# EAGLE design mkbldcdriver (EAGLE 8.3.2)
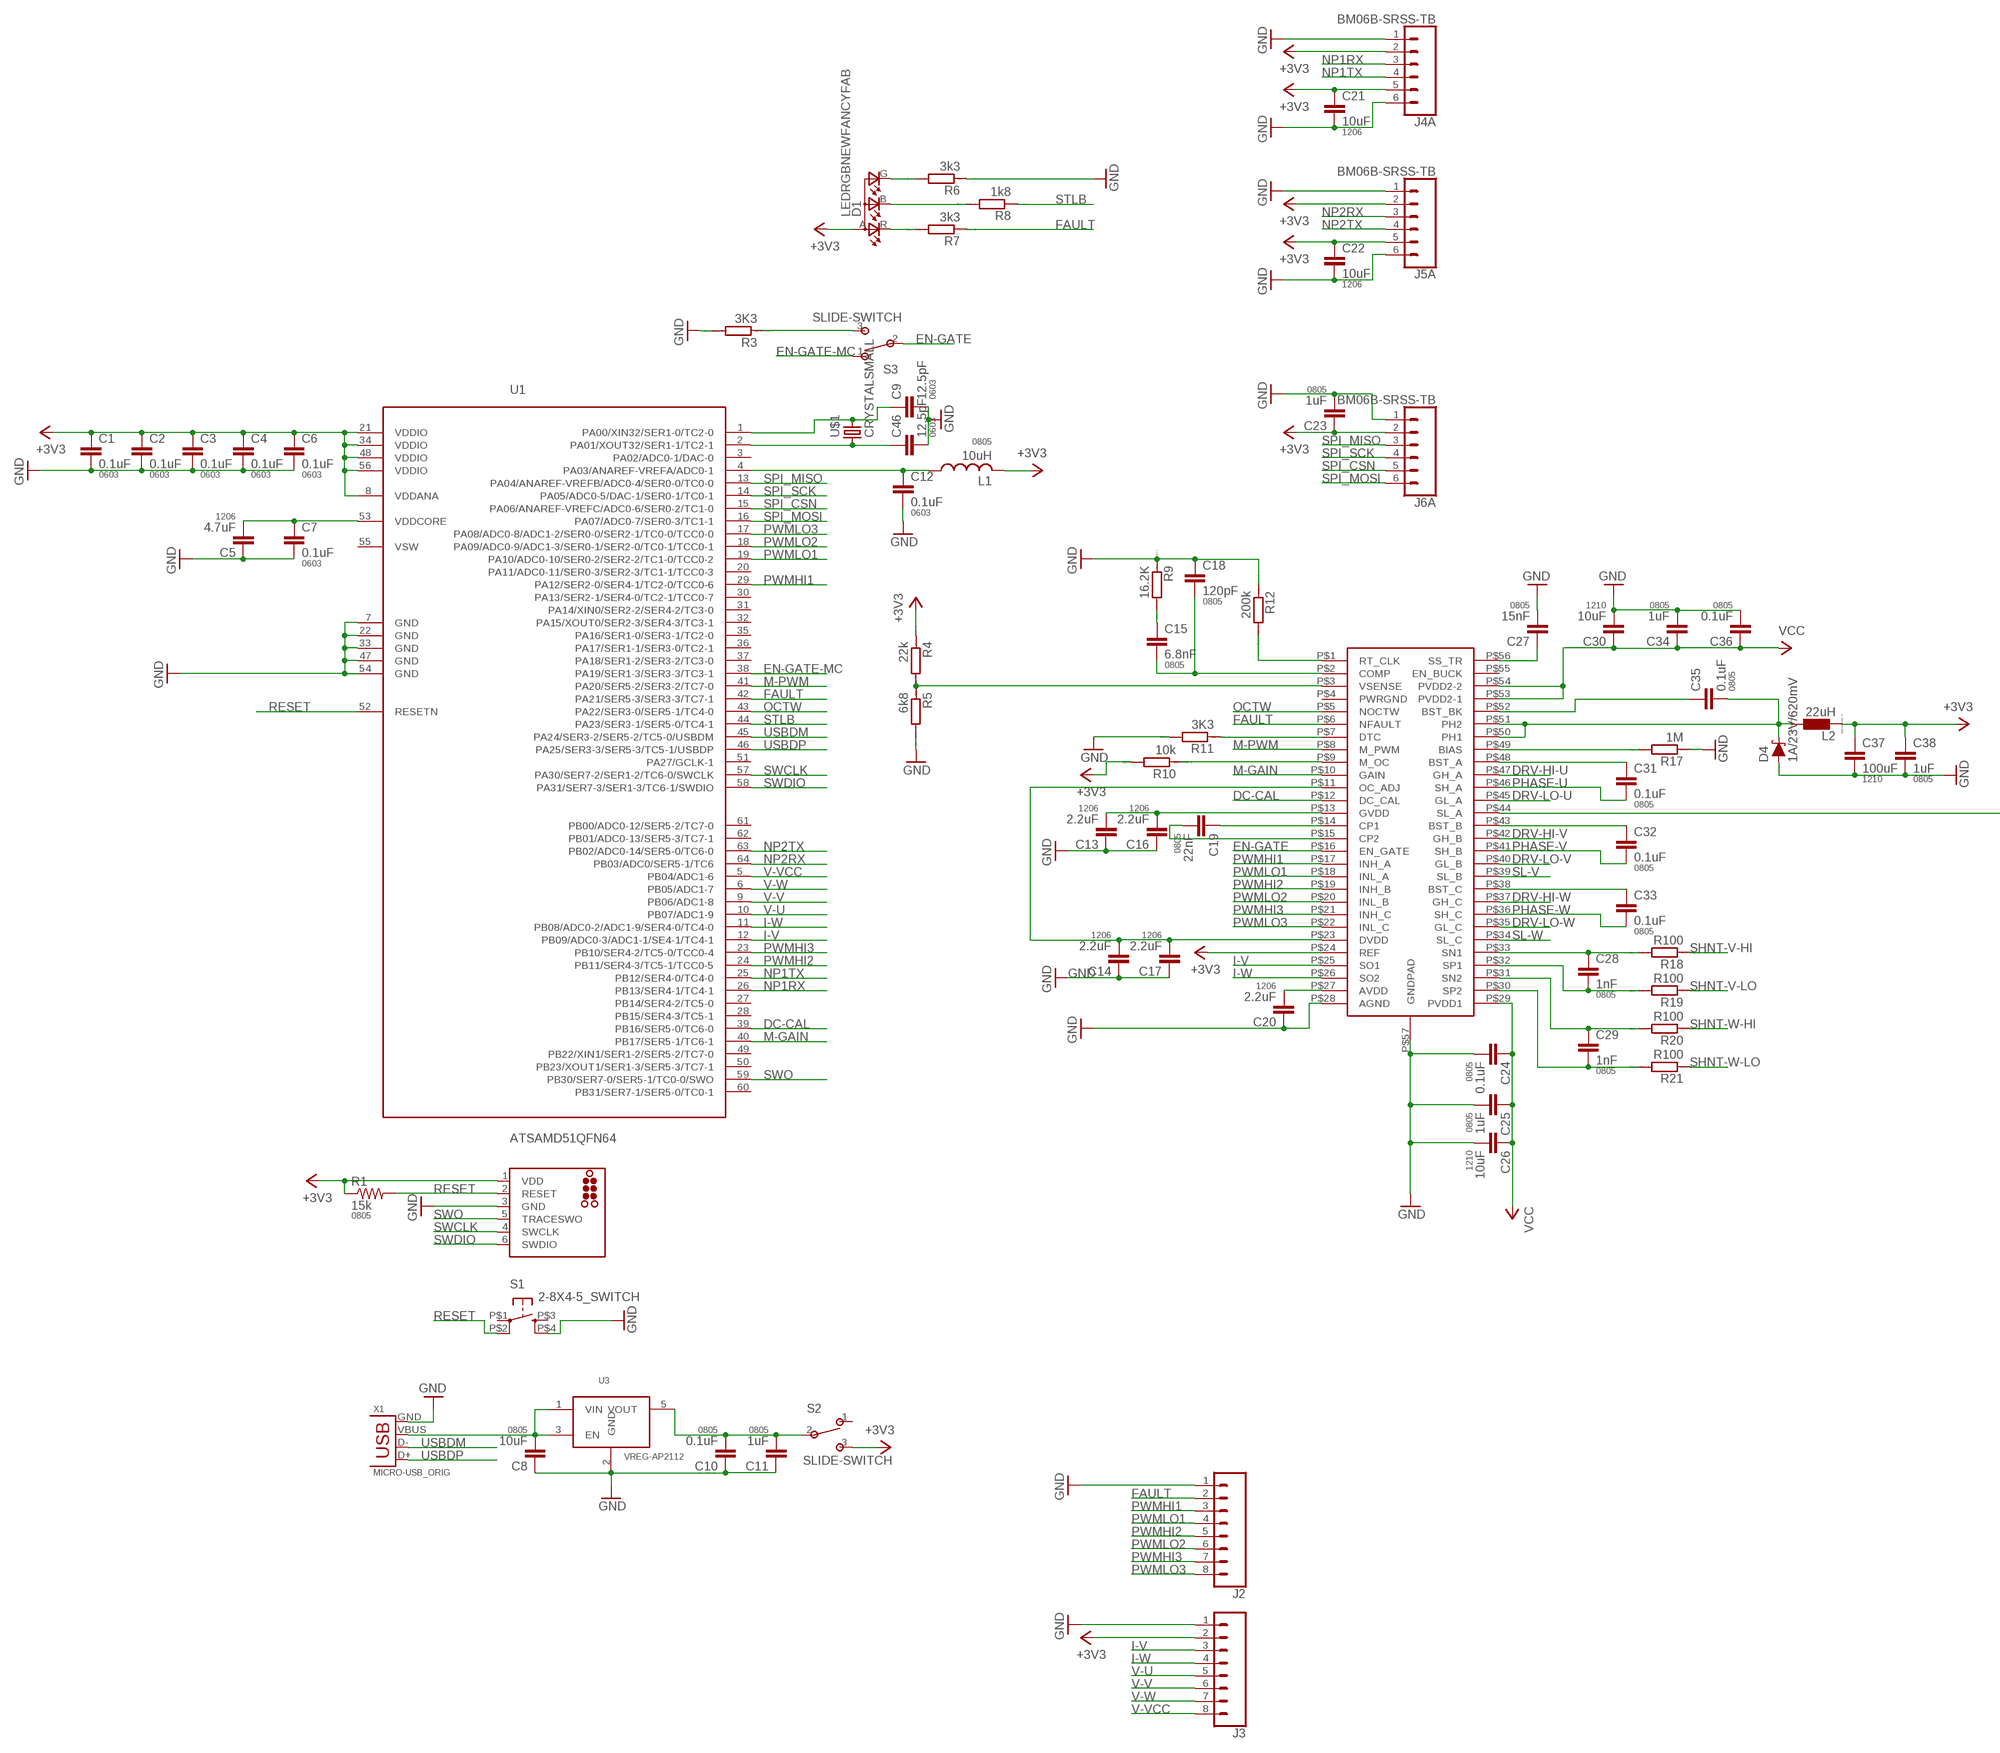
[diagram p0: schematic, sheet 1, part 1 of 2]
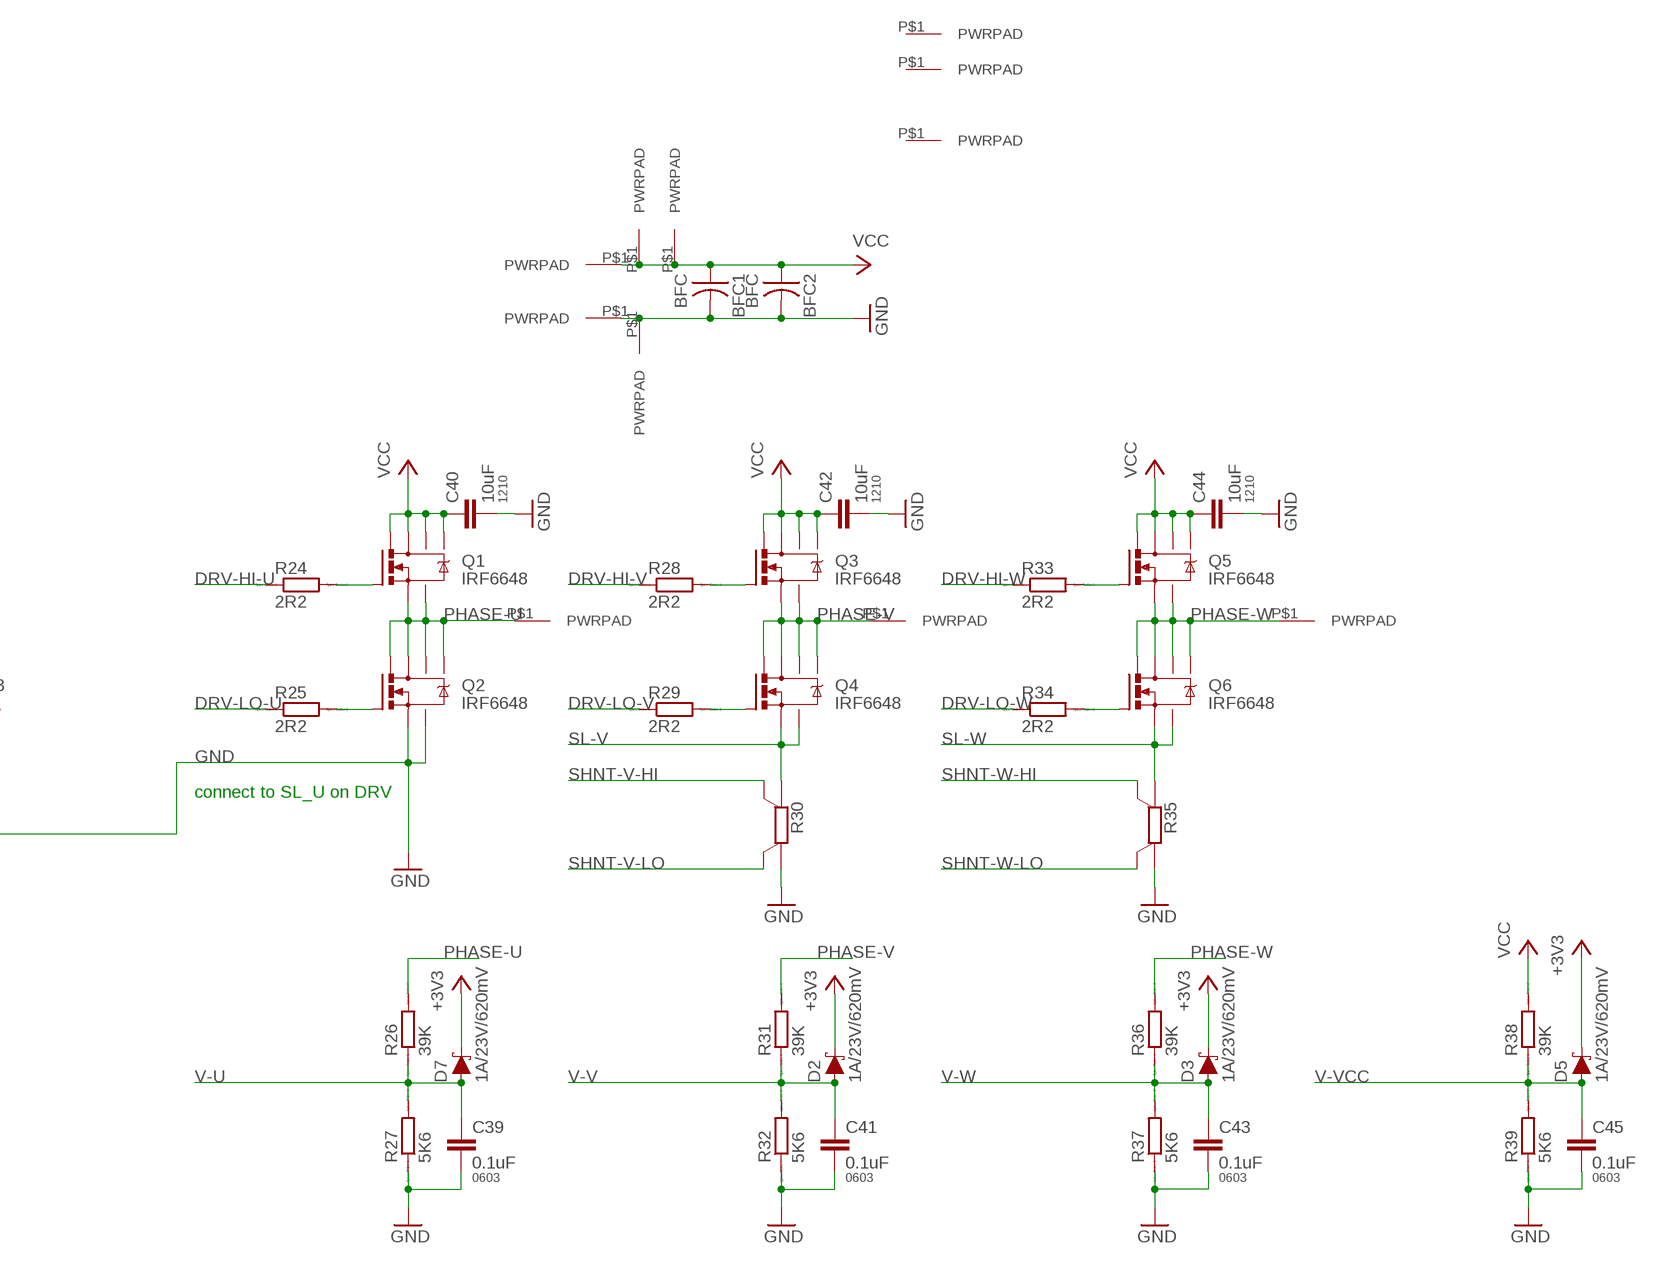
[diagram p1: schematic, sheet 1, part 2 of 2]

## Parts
BFC1  BFC  [BFC]
BFC2  BFC  [BFC]
C1  0.1uF  CAP0603-CAP  [0603-CAP]
C2  0.1uF  CAP0603-CAP  [0603-CAP]
C3  0.1uF  CAP0603-CAP  [0603-CAP]
C4  0.1uF  CAP0603-CAP  [0603-CAP]
C5  4.7uF  CAP1206  [1206]
C6  0.1uF  CAP0603-CAP  [0603-CAP]
C7  0.1uF  CAP0603-CAP  [0603-CAP]
C8  10uF  CAP0805  [0805]
C9  12.5pF  CAP0603-CAP  [0603-CAP]
C10  0.1uF  CAP0805  [0805]
C11  1uF  CAP0805  [0805]
C12  0.1uF  CAP0603-CAP  [0603-CAP]
C13  2.2uF  CAP1206  [1206]
C14  2.2uF  CAP1206  [1206]
C15  6.8nF  CAP0805  [0805]
C16  2.2uF  CAP1206  [1206]
C17  2.2uF  CAP1206  [1206]
C18  120pF  CAP0805  [0805]
C19  22nF  CAP0805  [0805]
C20  2.2uF  CAP1206  [1206]
C21  10uF  CAP1206  [1206]
C22  10uF  CAP1206  [1206]
C23  1uF  CAP0805  [0805]
C24  0.1uF  CAP0805  [0805]
C25  1uF  CAP0805  [0805]
C26  10uF  CAP1210  [1210]
C27  15nF  CAP0805  [0805]
C28  1nF  CAP0805  [0805]
C29  1nF  CAP0805  [0805]
C30  10uF  CAP1210  [1210]
C31  0.1uF  CAP0805  [0805]
C32  0.1uF  CAP0805  [0805]
C33  0.1uF  CAP0805  [0805]
C34  1uF  CAP0805  [0805]
C35  0.1uF  CAP0805  [0805]
C36  0.1uF  CAP0805  [0805]
C37  100uF  CAP1210  [1210]
C38  1uF  CAP0805  [0805]
C39  0.1uF  CAP0603-CAP  [0603-CAP]
C40  10uF  CAP1210  [1210]
C41  0.1uF  CAP0603-CAP  [0603-CAP]
C42  10uF  CAP1210  [1210]
C43  0.1uF  CAP0603-CAP  [0603-CAP]
C44  10uF  CAP1210  [1210]
C45  0.1uF  CAP0603-CAP  [0603-CAP]
C46  12.5pF  CAP0603-CAP  [0603-CAP]
D1  LEDRGBNEWFANCYFAB  [P-LCC-4-FANCYFAB]
D2  1A/23V/620mV  DIODE-SCHOTTKY-BAT20J  [SOD-323]
D3  1A/23V/620mV  DIODE-SCHOTTKY-BAT20J  [SOD-323]
D4  1A/23V/620mV  DIODE-SCHOTTKY-BAT20J  [SOD-323]
D5  1A/23V/620mV  DIODE-SCHOTTKY-BAT20J  [SOD-323]
D7  1A/23V/620mV  DIODE-SCHOTTKY-BAT20J  [SOD-323]
J1  TC2030-SWD-MCP  [TC2030-MCP]
J2  CONN_08NO_SILK_FEMALE_PTH  [1X08_NO_SILK]
J3  CONN_08NO_SILK_FEMALE_PTH  [1X08_NO_SILK]
J4  BM06B-SRSS-TB  JST_6_PIN_HORIZONTAL  [JST-6-SMD-HORI-1.0MM]
J5  BM06B-SRSS-TB  JST_6_PIN_HORIZONTAL  [JST-6-SMD-HORI-1.0MM]
J6  BM06B-SRSS-TB  JST_6_PIN_HORIZONTAL  [JST-6-SMD-HORI-1.0MM]
J7  PWRPAD2-5MM  [PWRPAD_2-5MM]
J8  PWRPADM3  [PWRPAD_3-25MM]
J9  PWRPADM3  [PWRPAD_3-25MM]
J10  PWRPADM3  [PWRPAD_3-25MM]
J11  PWRPADM3  [PWRPAD_3-25MM]
J12  PWRPADM3  [PWRPAD_3-25MM]
J13  PWRPADM3  [PWRPAD_3-25MM]
J14  PWRPADM3  [PWRPAD_3-25MM]
J15  PWRPADM3  [PWRPAD_3-25MM]
J16  PWRPAD2-5MM  [PWRPAD_2-5MM]
J17  PWRPAD2-5MM  [PWRPAD_2-5MM]
L1  10uH  INDUCTOR-0805  [0805]
L2  22uH  L  [L1812]
Q1  IRF6648  [DIRECTFET]
Q2  IRF6648  [DIRECTFET]
Q3  IRF6648  [DIRECTFET]
Q4  IRF6648  [DIRECTFET]
Q5  IRF6648  [DIRECTFET]
Q6  IRF6648  [DIRECTFET]
R1  15k  RESISTOR0805-RES  [0805]
R3  3K3  R  [R0805]
R4  22k  R  [R0805]
R5  6k8  R  [R0805]
R6  3k3  R  [R0805]
R7  3k3  R  [R0805]
R8  1k8  R  [R0805]
R9  16.2K  R  [R0805]
R10  10k  R  [R0805]
R11  3K3  R  [R0805]
R12  200k  R  [R0805]
R17  1M  R  [R0805]
R18  R100  R  [R0805]
R19  R100  R  [R0805]
R20  R100  R  [R0805]
R21  R100  R  [R0805]
R24  2R2  R  [R0805]
R25  2R2  R  [R0805]
R26  39K  R  [R0805]
R27  5K6  R  [R0805]
R28  2R2  R  [R0805]
R29  2R2  R  [R0805]
R30  WSL2726  [WSL2726]
R31  39K  R  [R0805]
R32  5K6  R  [R0805]
R33  2R2  R  [R0805]
R34  2R2  R  [R0805]
R35  WSL2726  [WSL2726]
R36  39K  R  [R0805]
R37  5K6  R  [R0805]
R38  39K  R  [R0805]
R39  5K6  R  [R0805]
S1  2-8X4-5_SWITCH  [TACT-SWITCH-KMR6]
S2  SLIDE-SWITCH  [AYZ0102AGRLC]
S3  SLIDE-SWITCH  [AYZ0102AGRLC]
U1  ATSAMD51QFN64  [QFN-64-9X9MM]
U2  DRV8302  [HTSSOP-56]
U3  VREG-AP2112  [SOT23-5]
U$1  CRYSTALSMALL  [2-SMD-1-5X3-2MM]
X1  MICRO-USB_ORIG  [DX4R005HJ5]

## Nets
+3V3: C1.1 C2.1 C3.1 C4.1 C6.1 C21.1 C22.1 C23.1 C37.1 C38.1 D1.A(A2) D2.C D3.C D5.C D7.C J1.1(VDD) J3.2 J4.2 J4.5 J5.2 J5.5 J6.2 L1.2 L2.2 R1.1 R4.1 R10.2 S2.3 U1.8(VDDANA) U1.21(VDDIO) U1.34(VDDIO) U1.48(VDDIO) U1.56(VDDIO) U2.P$24(REF)
CP1: C19.1 U2.P$14(CP1)
CP2: C19.2 U2.P$15(CP2)
DC-CAL: U1.39(PB16/SER5-0/TC6-0) U2.P$12(DC_CAL)
DRV-HI-U: R24.1 U2.P$47(GH_A)
DRV-HI-V: R28.1 U2.P$42(GH_B)
DRV-HI-W: R33.1 U2.P$37(GH_C)
DRV-LO-U: R25.1 U2.P$45(GL_A)
DRV-LO-V: R29.1 U2.P$40(GL_B)
DRV-LO-W: R34.1 U2.P$35(GL_C)
EN-GATE: S3.2 U2.P$16(EN_GATE)
EN-GATE-MC: S3.1 U1.38(PA19/SER1-3/SER3-3/TC3-1)
FAULT: J2.2 R7.1 U1.42(PA21/SER5-3/SER3-3/TC7-1) U2.P$6(NFAULT)
GND: BFC1.P$2 BFC2.P$2 C1.2 C2.2 C3.2 C4.2 C5.1 C6.2 C7.2 C8.1 C9.2 C10.1 C11.1 C12.2 C13.1 C14.1 C16.1 C17.1 C18.1 C20.1 C21.2 C22.2 C23.2 C24.2 C25.2 C26.2 C27.2 C30.2 C34.2 C36.2 C37.2 C38.2 C39.2 C40.2 C41.2 C42.2 C43.2 C44.2 C45.2 C46.2 D4.A J1.3(GND) J2.1 J3.1 J4.1 J4.6 J5.1 J5.6 J6.1 J9.P$1(PWRPAD) J11.P$1(PWRPAD) Q2.S@1(S) Q2.S@2(S) R3.2 R5.2 R6.1 R9.1 R11.2 R12.1 R17.1 R27.1 R30.A R32.1 R35.A R37.1 R39.1 S1.P$4(S1) U1.7(GND) U1.22(GND) U1.33(GND) U1.47(GND) U1.54(GND) U2.P$28(AGND) U2.P$44(SL_A) U2.P$57(GNDPAD) U3.2(GND) X1.GND
I-V: J3.3 U1.12(PB09/ADC0-3/ADC1-1/SE4-1/TC4-1) U2.P$25(SO1)
I-W: J3.4 U1.11(PB08/ADC0-2/ADC1-9/SER4-0/TC4-0) U2.P$26(SO2)
M-GAIN: U1.40(PB17/SER5-1/TC6-1) U2.P$10(GAIN)
M-PWM: U1.41(PA20/SER5-2/SER3-2/TC7-0) U2.P$8(M_PWM)
N$1: Q4.G R29.2
N$2: Q2.G R25.2
N$3: Q1.G R24.2
N$4: Q3.G R28.2
N$5: Q6.G R34.2
N$6: Q5.G R33.2
N$7: C33.1 U2.P$38(BST_C)
N$8: C32.1 U2.P$43(BST_B)
N$9: C31.1 U2.P$48(BST_A)
N$10: C27.1 U2.P$56(SS_TR)
N$11: C20.2 U2.P$27(AVDD)
N$12: C46.1 U1.2(PA01/XOUT32/SER1-1/TC2-1) U$1.P$1
N$13: C28.1 R18.2 U2.P$33(SN1)
N$14: C28.2 R19.2 U2.P$32(SP1)
N$15: C29.1 R20.2 U2.P$31(SN2)
N$16: C29.2 R21.2 U2.P$30(SP2)
N$17: C9.1 U1.1(PA00/XIN32/SER1-0/TC2-0) U$1.P$2
N$18: C13.2 C16.2 U2.P$13(GVDD)
N$19: C10.2 C11.2 S2.2 U3.5(VOUT)
N$20: C14.2 C17.2 U2.P$11(OC_ADJ) U2.P$23(DVDD)
N$21: R11.1 U2.P$7(DTC)
N$22: C8.2 U3.1(VIN) U3.3(EN) X1.VBUS
N$23: C35.1 U2.P$52(BST_BK)
N$24: R17.2 U2.P$49(BIAS)
N$25: R10.1 U2.P$9(M_OC)
N$26: R3.1 S3.3
N$27: C35.2 D4.C L2.1 U2.P$50(PH1) U2.P$51(PH2)
N$30: R12.2 U2.P$1(RT_CLK)
N$31: C15.2 C18.2 U2.P$2(COMP)
N$32: C15.1 R9.2
N$33: R4.2 R5.1 U2.P$3(VSENSE)
N$34: C12.1 L1.1 U1.4(PA03/ANAREF-VREFA/ADC0-1)
N$35: D1.G(CGREEN) R6.2
N$36: D1.B(CBLUE) R8.2
N$39: D1.R(CRED) R7.2
NP1RX: J4.3 U1.26(PB13/SER4-1/TC4-1)
NP1TX: J4.4 U1.25(PB12/SER4-0/TC4-0)
NP2RX: J5.3 U1.64(PB03/ADC0/SER5-1/TC6)
NP2TX: J5.4 U1.63(PB02/ADC0-14/SER5-0/TC6-0)
OCTW: U1.43(PA22/SER3-0/SER5-1/TC4-0) U2.P$5(NOCTW)
PHASE-U: C31.2 J7.P$1(PWRPAD) Q1.S@1(S) Q1.S@2(S) Q2.D@1(D) Q2.D@2(D) Q2.D@3(D) Q2.D@4(D) R26.2 U2.P$46(SH_A)
PHASE-V: C32.2 J16.P$1(PWRPAD) Q3.S@1(S) Q3.S@2(S) Q4.D@1(D) Q4.D@2(D) Q4.D@3(D) Q4.D@4(D) R31.2 U2.P$41(SH_B)
PHASE-W: C33.2 J17.P$1(PWRPAD) Q5.S@1(S) Q5.S@2(S) Q6.D@1(D) Q6.D@2(D) Q6.D@3(D) Q6.D@4(D) R36.2 U2.P$36(SH_C)
PWMHI1: J2.3 U1.29(PA12/SER2-0/SER4-1/TC2-0/TCC0-6) U2.P$17(INH_A)
PWMHI2: J2.5 U1.24(PB11/SER4-3/TC5-1/TCC0-5) U2.P$19(INH_B)
PWMHI3: J2.7 U1.23(PB10/SER4-2/TC5-0/TCC0-4) U2.P$21(INH_C)
PWMLO1: J2.4 U1.19(PA10/ADC0-10/SER0-2/SER2-2/TC1-0/TCC0-2) U2.P$18(INL_A)
PWMLO2: J2.6 U1.18(PA09/ADC0-9/ADC1-3/SER0-1/SER2-0/TC0-1/TCC0-1) U2.P$20(INL_B)
PWMLO3: J2.8 U1.17(PA08/ADC0-8/ADC1-2/SER0-0/SER2-1/TC0-0/TCC0-0) U2.P$22(INL_C)
RESET: J1.2(RESET) R1.2 S1.P$2(P1) U1.52(RESETN)
SHNT-V-HI: R18.1 R30.SB
SHNT-V-LO: R19.1 R30.SA
SHNT-W-HI: R20.1 R35.SB
SHNT-W-LO: R21.1 R35.SA
SL-V: Q4.S@1(S) Q4.S@2(S) R30.B U2.P$39(SL_B)
SL-W: Q6.S@1(S) Q6.S@2(S) R35.B U2.P$34(SL_C)
SPI_CSN: J6.5 U1.15(PA06/ANAREF-VREFC/ADC0-6/SER0-2/TC1-0)
SPI_MISO: J6.3 U1.13(PA04/ANAREF-VREFB/ADC0-4/SER0-0/TC0-0)
SPI_MOSI: J6.6 U1.16(PA07/ADC0-7/SER0-3/TC1-1)
SPI_SCK: J6.4 U1.14(PA05/ADC0-5/DAC-1/SER0-1/TC0-1)
STLB: R8.1 U1.44(PA23/SER3-1/SER5-0/TC4-1)
SWCLK: J1.4(SWCLK) U1.57(PA30/SER7-2/SER1-2/TC6-0/SWCLK)
SWDIO: J1.6(SWDIO) U1.58(PA31/SER7-3/SER1-3/TC6-1/SWDIO)
SWO: J1.5(TRACESWO) U1.59(PB30/SER7-0/SER5-1/TC0-0/SWO)
USBDM: U1.45(PA24/SER3-2/SER5-2/TC5-0/USBDM) X1.D-
USBDP: U1.46(PA25/SER3-3/SER5-3/TC5-1/USBDP) X1.D+
V-U: C39.1 D7.A J3.5 R26.1 R27.2 U1.10(PB07/ADC1-9)
V-V: C41.1 D2.A J3.6 R31.1 R32.2 U1.9(PB06/ADC1-8)
V-VCC: C45.1 D5.A J3.8 R38.1 R39.2 U1.5(PB04/ADC1-6)
V-W: C43.1 D3.A J3.7 R36.1 R37.2 U1.6(PB05/ADC1-7)
VCC: BFC1.P$1 BFC2.P$1 C24.1 C25.1 C26.1 C30.1 C34.1 C36.1 C40.1 C42.1 C44.1 J8.P$1(PWRPAD) J10.P$1(PWRPAD) J13.P$1(PWRPAD) Q1.D@1(D) Q1.D@2(D) Q1.D@3(D) Q1.D@4(D) Q3.D@1(D) Q3.D@2(D) Q3.D@3(D) Q3.D@4(D) Q5.D@1(D) Q5.D@2(D) Q5.D@3(D) Q5.D@4(D) R38.2 U2.P$29(PVDD1) U2.P$53(PVDD2-1) U2.P$54(PVDD2-2)
VDDCORE: C5.2 C7.1 U1.53(VDDCORE)
Unconnected: J4.M1 J4.M2 J5.M1 J5.M2 J6.M1 J6.M2 J12.P$1(PWRPAD) J14.P$1(PWRPAD) J15.P$1(PWRPAD) S1.P$1(P) S1.P$3(S) S2.1 U1.3(PA02/ADC0-1/DAC-0) U1.20(PA11/ADC0-11/SER0-3/SER2-3/TC1-1/TCC0-3) U1.27(PB14/SER4-2/TC5-0) U1.28(PB15/SER4-3/TC5-1) U1.30(PA13/SER2-1/SER4-0/TC2-1/TCC0-7) U1.31(PA14/XIN0/SER2-2/SER4-2/TC3-0) U1.32(PA15/XOUT0/SER2-3/SER4-3/TC3-1) U1.35(PA16/SER1-0/SER3-1/TC2-0) U1.36(PA17/SER1-1/SER3-0/TC2-1) U1.37(PA18/SER1-2/SER3-2/TC3-0) U1.49(PB22/XIN1/SER1-2/SER5-2/TC7-0) U1.50(PB23/XOUT1/SER1-3/SER5-3/TC7-1) U1.51(PA27/GCLK-1) U1.55(VSW) U1.60(PB31/SER7-1/SER5-0/TC0-1) U1.61(PB00/ADC0-12/SER5-2/TC7-0) U1.62(PB01/ADC0-13/SER5-3/TC7-1) U2.P$4(PWRGND) U2.P$55(EN_BUCK)

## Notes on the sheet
- connect to SL_U on DRV

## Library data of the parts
BFC1 BFC2 = fab:BFC
C1-C4 C6 C7 C9 C12 C39 C41 C43 C45 C46 = borkedlabs-passives:CAP: Capacitor; PACKAGE: 0603
C5 C13 C14 C16 C17 C20-C22 = borkedlabs-passives:CAP: Capacitor; PACKAGE: 1206
C8 C10 C11 C15 C18 C19 C23-C25 C27-C29 C31-C36 C38 = borkedlabs-passives:CAP: Capacitor; PACKAGE: 0805
C26 C30 C37 C40 C42 C44 = borkedlabs-passives:CAP: Capacitor; PACKAGE: 1210
D1 = fab:LEDRGBNEW
D2-D5 D7 = SparkFun-DiscreteSemi:DIODE-SCHOTTKY: Schottky diode; PROD_ID: DIO-11623
J1 = atsam:TC2030-SWD: TAG-CONNECT ICSP Connector Manufacturer: Tag-Connect Cable for easy In-Circuit Serial Programming. Designed for Microchip ICD2, suitable for many others. Two variants - one "with legs" (for hands-free fit on PCB) and another "without legs" for quick programming. PADDescription 1MCLR/Vpp 2Vdd 3GND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
J2 J3 = SparkFun-Connectors:CONN_08: Multi connection point. Often used as Generic Header-pin footprint for 0.1 inch spaced/style header connections On any of the 0.1 inch spaced packages, you can populate with these: Break Away Headers - Straight (PRT-00116) Break Away Male Headers - Right Angle (PRT-00553) Female Headers (PRT-00115)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; PROD_ID: CONN-08438
J4-J6 = SparkFun-Connectors:JST_6_PIN_HORIZONTAL: JST 6 pin horizontal connector JST-SH type. Here is the connector we sell at SparkFun: name (XXX-00000) Datasheet It was used on these SparkFun products: name (XXX-00000) name (XXX-00000); PROD_ID: XXX-00000
J7 J16 J17 = fab:PWRPAD
J8-J15 = power:PWRPAD
L1 = borkedlabs-passives:INDUCTOR; PACKAGE: 0805
L2 = eagle-ltspice:L: INDUCTOR, European symbol; SPICEMODEL: NONE; SPICEPREFIX: L
Q1-Q6 = transistor-power:IRF6648: DirectFET Power MOSFET Source: http://www.irf.com/product-info/datasheets/data/irf6648.pdf
R1 = borkedlabs-passives:RESISTOR: Resistor; PACKAGE: 0805
R3-R12 R17-R21 R24-R29 R31-R34 R36-R39 = eagle-ltspice:R: RESISTOR, European symbol; SPICEMODEL: NONE; SPICEPREFIX: R
R30 R35 = fab:WSL2726: SMD SHUNT RESISTOR
S1 = fab:2-8X4-5_SWITCH
S2 S3 = fab:SLIDE-SWITCH: SMD slide-switch AYZ0102AGRLC as found in the fablab inventory. Includes the mounting holes. Made by Zaerc.
U1 = atsam:ATSAMD51
U2 = power:DRV8302
U3 = power:VREG-AP2112
U$1 = fab:CRYSTAL
X1 = fab:MICRO-USB: SMD micro USB connector as found in the fablab inventory. Three footprint variants included: original, as described by manufacturer's datasheet for milling with the 1/100" bit for milling with the 1/64" bit Made by Zaerc.

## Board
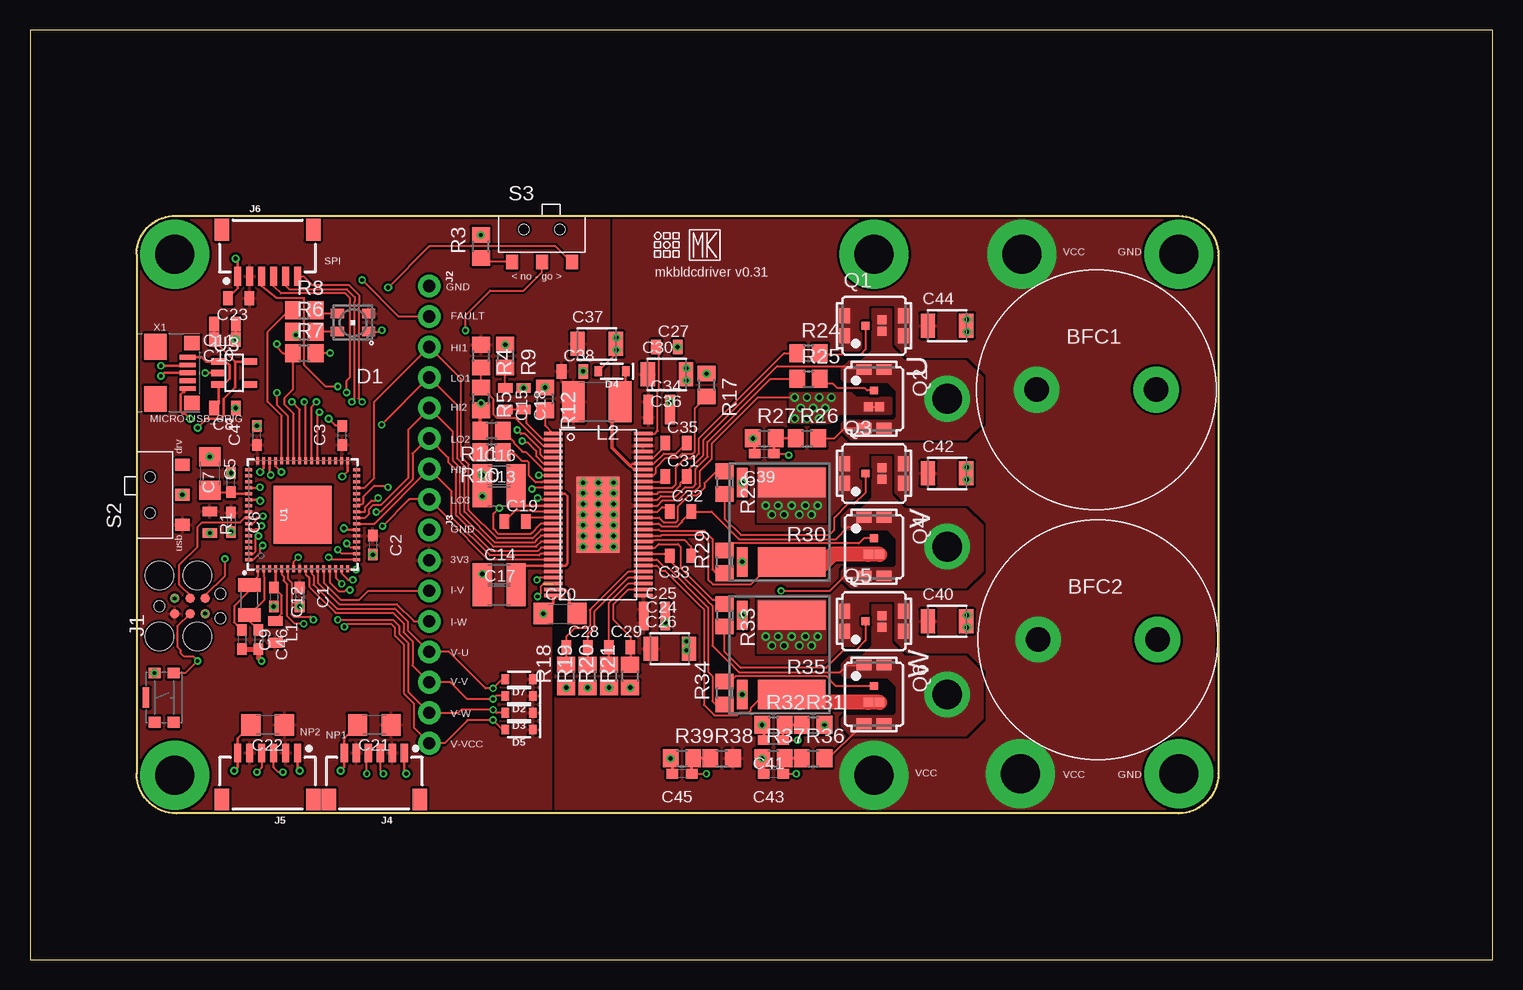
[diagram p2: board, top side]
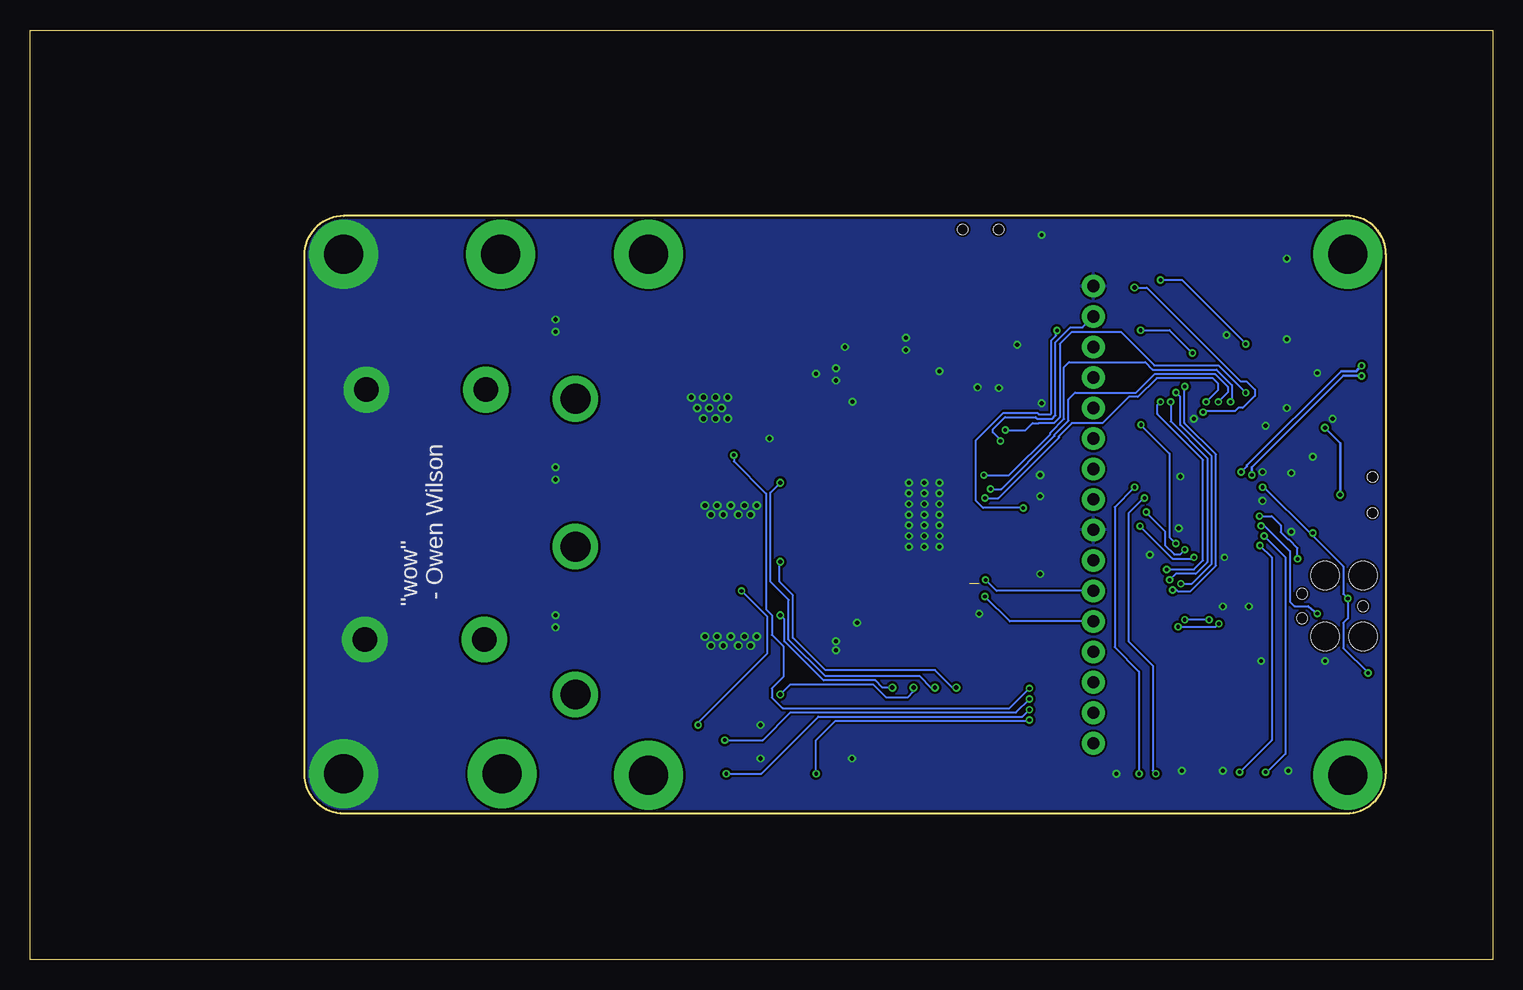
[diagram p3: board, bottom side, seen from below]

Size 121.92 x 77.47 mm. Coordinates in mm from the lower left corner, seen from the top.
Outline: 0,0 121.92,0 121.92,77.47 0,77.47 0,0
Outline: 8.89,58.8 8.89,15.49 arc90 12.19,12.19 95.76,12.19 arc90 99.06,15.49 99.06,58.67 arc90 95.76,61.98 12.19,61.98 arc92 8.89,58.8
Copper layers (1*16): Top 0.035mm / dielectric 1.5mm / Bottom 0.035mm
Design rules "default *": minimum track width 6mil, minimum drill 0.3mm, track to track 8mil, track to pad 8mil, pad to pad 8mil, via to via 8mil, smd to smd 8mil, copper to edge 8mil, drill to drill 8mil, minimum pad ring 10mil, minimum via ring 6mil, stop-mask expansion 4mil, vias tented up to drill 20mil, thermal gap 8mil

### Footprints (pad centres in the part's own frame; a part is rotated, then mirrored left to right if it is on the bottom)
BFC = drill 2.032 pad 3.81: P$1 -4.978,0; P$2 4.978,0
0603-CAP = smd 0.96 x 0.8: 1 -0.8,0; 2 0.8,0
1206 = smd 1.6 x 1.8: 1 -1.4,0; 2 1.4,0
0805 = smd 0.8 x 1.2: 1 -0.9,0; 2 0.9,0
1210 = smd 1.2 x 2: 1 -1.6,0; 2 1.6,0
P-LCC-4-FANCYFAB = smd 0.8 x 1.1: A 0.75,-1.3; B 0.75,1.3; G -0.75,1.3; R -0.75,-1.3
SOD-323 = smd 0.63 x 0.83: A 1.15,0; C -1.15,0
TC2030-MCP = smd 0.787 x 0.787: 1 1.27,-0.635; 2 1.27,0.635; 3 2.54,-0.635; 4 2.54,0.635; 5 3.81,-0.635; 6 3.81,0.635 | hole 0.889: 0,0; 5.08,-1.016; 5.08,1.016 | hole 2.375: 0,2.54; 0,-2.54; 3.175,-2.54; 3.175,2.54
1X08_NO_SILK = drill 1.016 pad 1.88: 1 0,0; 2 2.54,0; 3 5.08,0; 4 7.62,0; 5 10.16,0; 6 12.7,0; 7 15.24,0; 8 17.78,0
JST-6-SMD-HORI-1.0MM = smd 0.6 x 1.55: 1 -2.5,-4.775; 2 -1.5,-4.775; 3 -0.5,-4.775; 4 0.5,-4.775; 5 1.5,-4.775; 6 2.5,-4.775 | smd 1.2 x 1.8: M1 -3.8,-0.9; M2 3.8,-0.9
PWRPAD_2-5MM = drill 2.489 pad 3.81: P$1 0,0
PWRPAD_3-25MM = drill 3.25 pad 5.75: P$1 0,0
L1812 = smd 1.9 x 3.4: 1 -1.95,0; 2 1.95,0
DIRECTFET = smd 0.9 x 1.25: D@1 -2.45,0.825; D@2 -2.45,-0.825; D@3 2.45,0.825; D@4 2.45,-0.825 | smd 0.65 x 0.65: G -0.7,0 | smd 0.75 x 0.75: S@1 0.65,0.475; S@2 0.65,-0.475
R0805 = smd 1.3 x 1.5: 1 -0.95,0; 2 0.95,0
WSL2726 = smd 2.438 x 5.588: A 3.302,2.794; B -3.302,2.794 | smd 2.438 x 0.889: SA 3.302,6.921; SB -3.302,6.921
TACT-SWITCH-KMR6 = smd 0.9 x 1: P$1 -2.05,0.8; P$2 2.05,0.8; P$3 -2.05,-0.8; P$4 2.05,-0.8 | smd 1.7 x 0.55: P$5 0,1.5
AYZ0102AGRLC = smd 1 x 1.2: 1 2.5,-2.3; 2 0,-2.3; 3 -2.5,-2.3 | hole 0.85: -1.5,0.4; 1.5,0.4
QFN-64-9X9MM = smd 0.6 x 0.25: 1 -4.5,3.75; 2 -4.5,3.25; 3 -4.5,2.75; 4 -4.5,2.25; 5 -4.5,1.75; 6 -4.5,1.25; 7 -4.5,0.75; 8 -4.5,0.25; 9 -4.5,-0.25; 10 -4.5,-0.75; 11 -4.5,-1.25; 12 -4.5,-1.75; 13 -4.5,-2.25; 14 -4.5,-2.75; 15 -4.5,-3.25; 16 -4.5,-3.75; 33 4.5,-3.75; 34 4.5,-3.25; 35 4.5,-2.75; 36 4.5,-2.25; 37 4.5,-1.75; 38 4.5,-1.25; 39 4.5,-0.75; 40 4.5,-0.25; 41 4.5,0.25; 42 4.5,0.75; 43 4.5,1.25; 44 4.5,1.75; 45 4.5,2.25; 46 4.5,2.75; 47 4.5,3.25; 48 4.5,3.75 | smd 0.25 x 0.6: 17 -3.75,-4.5; 18 -3.25,-4.5; 19 -2.75,-4.5; 20 -2.25,-4.5; 21 -1.75,-4.5; 22 -1.25,-4.5; 23 -0.75,-4.5; 24 -0.25,-4.5; 25 0.25,-4.5; 26 0.75,-4.5; 27 1.25,-4.5; 28 1.75,-4.5; 29 2.25,-4.5; 30 2.75,-4.5; 31 3.25,-4.5; 32 3.75,-4.5; 49 3.75,4.5; 50 3.25,4.5; 51 2.75,4.5; 52 2.25,4.5; 53 1.75,4.5; 54 1.25,4.5; 55 0.75,4.5; 56 0.25,4.5; 57 -0.25,4.5; 58 -0.75,4.5; 59 -1.25,4.5; 60 -1.75,4.5; 61 -2.25,4.5; 62 -2.75,4.5; 63 -3.25,4.5; 64 -3.75,4.5 | smd 4.826 x 4.826: P$1 0,0
HTSSOP-56 = smd 1.549 x 0.279: P$1 -3.75,6.75; P$2 -3.75,6.25; P$3 -3.75,5.75; P$4 -3.75,5.25; P$5 -3.75,4.75; P$6 -3.75,4.25; P$7 -3.75,3.75; P$8 -3.75,3.25; P$9 -3.75,2.75; P$10 -3.75,2.25; P$11 -3.75,1.75; P$12 -3.75,1.25; P$13 -3.75,0.75; P$14 -3.75,0.25; P$15 -3.75,-0.25; P$16 -3.75,-0.75; P$17 -3.75,-1.25; P$18 -3.75,-1.75; P$19 -3.75,-2.25; P$20 -3.75,-2.75; P$21 -3.75,-3.25; P$22 -3.75,-3.75; P$23 -3.75,-4.25; P$24 -3.75,-4.75; P$25 -3.75,-5.25; P$26 -3.75,-5.75; P$27 -3.75,-6.25; P$28 -3.75,-6.75; P$29 3.75,-6.75; P$30 3.75,-6.25; P$31 3.75,-5.75; P$32 3.75,-5.25; P$33 3.75,-4.75; P$34 3.75,-4.25; P$35 3.75,-3.75; P$36 3.75,-3.25; P$37 3.75,-2.75; P$38 3.75,-2.25; P$39 3.75,-1.75; P$40 3.75,-1.25; P$41 3.75,-0.75; P$42 3.75,-0.25; P$43 3.75,0.25; P$44 3.75,0.75; P$45 3.75,1.25; P$46 3.75,1.75; P$47 3.75,2.25; P$48 3.75,2.75; P$49 3.75,3.25; P$50 3.75,3.75; P$51 3.75,4.25; P$52 3.75,4.75; P$53 3.75,5.25; P$54 3.75,5.75; P$55 3.75,6.25; P$56 3.75,6.75 | smd 3.581 x 6.35: P$57 0,0
SOT23-5 = smd 0.533 x 1.194: 1 -0.95,-1.306; 2 0,-1.306; 3 0.95,-1.306; 4 0.95,1.306; 5 -0.95,1.306
2-SMD-1-5X3-2MM = smd 1.1 x 1.9: P$1 -1.25,0; P$2 1.25,0
DX4R005HJ5 = smd 0.4 x 1.35: D+ 0,1.6; D- -0.65,1.6; GND 1.3,1.6; ID 0.65,1.6; VBUS -1.3,1.6 | smd 1.2 x 1.3: GND@1 -2.5,1.95; GND@2 2.5,1.95 | smd 2.15 x 1.9: GND@3 -2.175,-1.1; GND@4 2.175,-1.1

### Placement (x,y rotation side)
BFC1  88.9,47.5 0 top
BFC2  89.03,26.67 0 top
C1  22.48,30.23 270 top
C2  28.57,34.54 270 top
C3  26.04,43.69 90 top
C4  18.92,43.69 90 top
C5  14.99,40.51 270 top
C6  16.76,36.45 270 top
C7  16.76,39.75 90 top
C8  16.26,45.97 180 top
C9  17.65,26.67 270 top
C10  16.26,51.69 180 top
C11  16.26,52.96 180 top
C12  20.32,30.23 270 top
C13  39.12,38.61 0 top
C14  39.12,32.13 0 top
C15  39.62,46.74 270 top
C16  39.12,40.39 0 top
C17  39.12,30.35 0 top
C18  41.15,46.74 270 top
C19  40.45,36.51 0 top
C20  44.2,28.83 0 top
C21  28.7,19.56 180 top
C22  19.81,19.56 180 top
C23  17.4,55.12 180 top
C24  52.07,28.07 0 top
C25  52.07,29.21 0 top
C26  53.34,25.91 0 top
C27  53.09,51.05 0 top
C28  45.59,26.04 0 top
C29  49.15,26.04 0 top
C30  53.09,48.77 0 top
C31  53.85,40.26 0 top
C32  54.23,37.34 0 top
C33  54.23,33.66 180 top
C34  52.45,46.48 0 top
C35  53.85,43.05 0 top
C36  52.45,45.21 0 top
C37  47.24,51.31 0 top
C38  45.21,49.02 0 top
C39  61.21,42.16 180 top
C40  76.45,28.19 0 top
C41  61.98,18.29 180 top
C42  76.45,40.51 0 top
C43  61.98,15.49 180 top
C44  76.45,52.83 0 top
C45  54.36,15.49 180 top
C46  19.05,26.67 270 top
D1  26.92,53.09 90 top
D2  40.77,21.97 180 top
D3  40.77,20.57 180 top
D4  48.51,49.02 180 top
D5  40.77,19.18 180 top
D7  40.77,23.37 180 top
J1  10.79,29.46 0 top
J2  33.27,56.13 270 top
J3  33.27,35.81 270 top
J4  28.7,12.45 180 top
J5  19.81,12.45 180 top
J6  19.81,61.72 0 top
J7  76.45,46.74 0 top
J8  82.68,58.8 0 top
J9  95.76,58.8 0 top
J10  82.55,15.49 0 top
J11  95.76,15.49 0 top
J12  70.36,58.8 0 top
J13  70.36,15.37 0 top
J14  12.06,58.8 0 top
J15  12.06,15.37 0 top
J16  76.45,34.42 0 top
J17  76.45,22.1 0 top
L1  20.45,27.3 270 top
L2  47.24,46.48 180 top
Q1  70.36,52.83 0 top
Q2  70.36,46.74 270 top
Q3  70.36,40.51 0 top
Q4  70.36,34.42 270 top
Q5  70.36,28.19 0 top
Q6  70.36,22.1 270 top
R1  14.99,36.45 270 top
R3  37.59,59.44 90 top
R4  37.59,50.29 270 top
R5  37.59,46.74 270 top
R6  22.86,52.32 0 top
R7  22.86,50.55 0 top
R8  22.86,54.1 0 top
R9  39.62,50.29 270 top
R10  38.48,42.29 180 top
R11  38.48,44.07 180 top
R12  42.93,46.74 270 top
R17  56.39,47.88 270 top
R18  44.7,23.62 90 top
R19  46.48,23.62 90 top
R20  48.26,23.62 90 top
R21  50.04,23.62 90 top
R24  64.9,50.55 0 top
R25  64.9,48.39 0 top
R26  64.77,43.43 0 top
R27  61.21,43.43 0 top
R28  57.91,39.75 270 top
R29  57.91,33.15 90 top
R30  66.29,36.45 90 top
R31  65.28,19.56 0 top
R32  61.98,19.56 0 top
R33  57.91,28.7 270 top
R34  57.91,22.23 90 top
R35  66.29,25.4 90 top
R36  65.28,16.76 0 top
R37  61.98,16.76 0 top
R38  57.66,16.76 0 top
R39  54.36,16.76 0 top
S1  11.18,21.84 90 top
S2  10.41,38.73 90 top
S3  42.67,60.45 0 top
U1  22.73,37.08 90 top
U2  47.37,37.08 0 top
U3  17.02,48.9 270 top
U$1  18.29,29.97 90 top
U$2  [CBA-SILK-LOGO]  53.09,59.56 0 top
U$3  [MK-LOGO-SILK]  56.26,59.56 0 top
X1  11.56,48.9 270 top

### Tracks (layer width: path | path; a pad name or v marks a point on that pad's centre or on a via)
+3V3
  pour Top: 48.26,61.98 48.26,44.2 43.43,44.2 43.43,12.19 8.89,12.19 8.89,61.98
CP1
  Top 0.152: U2.P$14 41.92,37.33 41.87,37.39 40.43,37.39 C19.1
CP2
  Top 0.152: U2.P$15 41.67,36.83 C19.2
DC-CAL  (via drill 0.3)
  Top 0.152: U2.P$12 42.45,38.33 v42.32,38.47 | U1.39 23.48,46.09 v23.88,46.48
  Bottom 0.152: v42.32,38.47 41.2,38.47 36.16,43.5 36.16,43.61 35.07,44.7 32.51,44.7 30.33,46.89 29.57,46.89 28,48.46 23.32,48.46 22.86,48.01 22.86,47.5 v23.88,46.48
DRV-HI-U
  Top 0.152: U2.P$47 53.56,39.33 53.85,39.62 53.85,41.02 54.61,41.78 55.38,41.78 55.78,42.19 55.78,43.46 62.87,50.55 R24.1
DRV-HI-V
  Top 0.152: U2.P$42 52.44,36.83 52.81,36.46 53.84,36.46 54.01,36.62 54.01,37.76 54.91,38.66 55.55,38.66 56.21,39.32 56.21,39.7 57.21,40.7 R28.1 57.66,40.57
DRV-HI-W
  Top 0.152: U2.P$37 52.11,34.33 52.4,34.62 54.02,34.62 54.23,34.42 54.23,32.64 56.9,29.97 57.59,29.97 R33.1
DRV-LO-U
  Top 0.152: U2.P$45 52.31,38.33 52.6,38.62 53.86,38.62 54.61,39.37 55.25,39.37 55.43,39.54 55.43,39.55 55.5,39.62 55.5,40.9 56.49,41.9 56.49,43.17 56.5,43.17 61.72,48.39 R25.1
DRV-LO-V
  Top 0.152: U2.P$40 52.43,35.83 52.52,35.75 56.2,35.75 56.9,35.05 56.9,34.88 56.88,34.86 56.88,32.52 57.15,32.26 57.85,32.26 R29.1
DRV-LO-W
  Top 0.152: R34.1 57.15,21.27 56.88,21.54 56.88,23.64 56.53,23.99 56.53,29.33 56.16,29.7 53.09,32.78 52.81,32.78 52.26,33.33 U2.P$35
EN-GATE  (via drill 0.3)
  Top 0.152: v36.31,52.44 36.31,53.71 38.35,55.75 41.15,55.75 42.67,57.28 S3.2 | U2.P$16 42.58,36.33 41.8,35.55 41.72,35.47 41.59,35.47 39.08,35.47 38.64,35.91 38.64,37.16 v39.12,37.64
  Bottom 0.152: v36.31,52.44 36.38,52.36 36.38,52 36.78,51.61 36.78,45.51 36.85,45.44 37.82,45.44 37.95,45.57 40.79,45.57 43.05,43.3 43.05,38.23 42.47,37.64 v39.12,37.64
EN-GATE-MC  (via drill 0.3, 0.35)
  Top 0.152: S3.1 45.1,58.15 43.81,59.44 33.27,59.44 v29.84,56.01 | U1.38 23.98,45.48 v24.13,45.62
  Bottom 0.152: v29.84,56.01 28.83,56.01 21.02,48.19 20.51,48.19 19.81,47.5 19.81,46.99 20.83,45.97 21.21,45.97 21.46,45.72 24.03,45.72 v24.13,45.62
FAULT  (via drill 0.3)
  Top 0.152: U2.P$6 42.81,41.33 42.21,41.93 42.21,42.37 42.16,42.42 42.16,42.43 41.53,43.06 41.18,43.06 v41.03,43.21 | U1.42 21.98,45.48 21.24,46.23 21.24,46.84 21.91,47.51 R7.1 21.08,50.55 20.57,51.05 v20.57,51.31 | J2.2 30.73,53.59 v27.69,56.64
  Bottom 0.152: v41.03,43.21 41.03,43.31 41.66,43.94 41.66,44.2 40.64,45.21 38.1,45.21 37.96,45.07 37.95,45.08 36.71,45.08 36.42,45.36 36.42,51.46 35.31,52.58 35.3,52.58 35.2,52.68 34.19,52.68 J2.2 | v27.69,56.64 25.91,56.64 v20.57,51.31
GND  (via drill 0.3, 0.35, 0.4)
  Top 0.152: C17.1 C14.1 | U2.P$44 52.31,37.83 52.75,38.27 54.01,38.27 54.76,39.01 55.4,39.01 55.85,39.47 55.85,40.75 56.85,41.75 56.85,43.01 60.7,46.86 v63.75,46.86 | R6.1 v22.18,52.05 | U1.7 21.98,33.16 v22.35,33.53 | S1.P$4 12.97,23.89 v13.97,24.89 13.59,25.27 12.83,25.27 12.57,25.53 12.57,25.78 12.32,26.04 12.32,27.81 J1.3
  Top 0.203: 48.78,37.83 v48.64,37.97 | Q2.S@2 Q2.S@1 | U1.54 19.07,38.33 v19.18,38.23 | U1.47 19.48,40.95 v19.18,40.64 | U1.33 26.48,40.71 v26.04,40.26 | U1.22 26.27,35.83 v26.16,35.94 | X1.GND 12.86,47.3 12.73,47.3 12.55,47.12 12.55,45.67 12.73,45.49 12.93,45.49 v13.34,45.09 | C11.1 C10.1 | v17.14,58.42 17.31,58.25 J6.1 17.31,55.93 C23.2 | C22.2 17.31,18.46 J5.6 17.31,16.04 v17.02,15.75 | C21.2 26.2,18.46 J4.6 26.2,16.04 v25.91,15.75 | J5.1 22.31,15.91 v22.48,15.75 | J4.1 31.2,15.66 v31.37,15.49 | C39.2 60.36,43.33 R27.1 | v78.11,53.34 78.05,53.29 C44.2 78.05,52.38 v78.11,52.32 | v78.11,41.02 78.05,40.97 C42.2 78.05,40.06 v78.11,40.01 | v78.11,28.7 78.05,28.65 C40.2 78.05,27.74 v78.11,27.69 | C41.2 61.13,19.46 R32.1 | C43.2 61.13,16.66 R37.1 | C45.2 53.51,16.66 R39.1 | C3.2 25.44,44.54 v24.89,45.09 | U3.2 v14.61,48.9 | C37.2 48.84,50.5 D4.A
  Top 0.254: U2.P$28 43.62,29.65 C20.1
  Top 0.305: R11.2 37.53,45.73 R5.2 v37.59,46.35 | v48.9,51.82 48.84,51.77 C37.2 48.84,50.85 v48.9,50.8 | C36.2 C34.2 | v54.74,49.28 54.69,49.23 C30.2 54.69,48.31 v54.74,48.26 | C25.2 C24.2 | v54.74,26.54 54.69,26.11 C26.2 54.69,25.2 v54.74,25.78
  Top 0.406: C9.2 C46.2 19.05,25.15 v19.3,24.89
  other vias: 46.1,39.75 47.37,39.75 48.64,39.75 46.1,38.86 46.1,37.97 46.1,37.08 46.1,35.31 46.1,36.2 46.1,34.42 47.37,38.86 47.37,37.97 48.64,38.86 48.64,37.08 47.37,37.08 47.37,36.2 47.37,35.31 47.37,34.42 48.64,36.2 48.64,35.31 48.64,34.42 37.72,40.39 65.66,26.92 64.64,26.92 63.5,26.92 62.36,26.92 61.34,26.92 61.85,26.16 64.64,37.85 63.5,37.85 65.66,37.85 61.85,37.08 62.36,37.85 65.15,37.08 61.34,37.85 62.87,37.08 64.14,37.08 63.75,45.09 64.77,46.86 64.26,45.97 66.8,46.86 66.29,45.97 65.79,45.09 64.77,45.09 65.28,45.97 65.79,46.86 65.15,26.16 62.87,26.16 64.14,26.16 42.93,47.69 41.15,47.64 39.62,51.24 37.72,38.61 42.8,28.83 28.57,33.74 16.76,35.65 14.99,41.91 16.76,40.55 18.92,44.49 17.16,45.97 17.16,51.69 22.48,29.43 20.32,29.43 37.72,32.13 46.11,49.02 53.99,51.05 56.39,48.83 53.35,46.48 52.97,28.07 37.59,60.39 60.26,43.43 61.03,19.56 61.03,16.76 53.41,16.76
  pour Bottom: 8.89,61.98 99.06,61.98 99.06,12.19 8.89,12.19
  pour Top (isolate 0.254, no thermals): 68.83,46.86 71.75,46.86 71.75,45.47 67.44,45.47 66.67,44.7 63.37,44.7 63.37,47.24 68.45,47.24
  pour Top (no thermals): 60.71,36.45 60.71,41.02 66.29,41.02 66.29,36.45
  pour Top (no thermals): 60.71,25.53 60.71,29.97 66.29,29.97 66.29,25.53
  pour Top (rank 3, no thermals): 43.56,44.07 43.56,30.1 50.29,30.1 50.29,40.89 48.51,42.67 48.51,44.07
I-V  (via drill 0.3)
  Top 0.152: J3.3 28.19,30.73 27.43,29.97 25.91,29.97 24.48,31.4 U1.12 | U2.P$25 42.45,31.83 v42.27,31.65
  Bottom 0.152: J3.3 41.35,30.73 v42.27,31.65
I-W  (via drill 0.3)  (1 unrouted)
  Top 0.152: v42.31,30.26 42.57,30.51 42.57,31.09 42.81,31.33 | J3.4 32,28.19 30.58,29.62 25.76,29.62 24.64,30.73 23.98,31.39 U1.11
  Bottom 0.152: J3.4 40.25,28.19 v42.31,30.26
M-GAIN  (via drill 0.3)
  Top 0.152: U2.P$10 41.97,39.33 v41.85,39.21 | U1.40 22.98,46.36 v22.86,46.48
  Bottom 0.152: v41.85,39.21 40.95,39.21 36.52,43.65 36.52,43.76 35.36,44.92 35.36,46.69 34.8,47.24 29.72,47.24 28.14,48.82 23.16,48.82 23.11,48.77 23.11,48.76 22.07,47.72 22.07,47.27 v22.86,46.48
M-PWM  (via drill 0.3)
  Top 0.152: U2.P$8 42.45,40.33 v42.41,40.37 | U1.41 22.48,45.84 v21.84,46.48
  Bottom 0.152: v42.41,40.37 40.3,40.37 36.87,43.8 36.87,43.9 35.71,45.06 35.71,49.38 35.31,49.78 28.95,49.78 28.34,49.17 23.01,49.17 21.71,47.88 21.71,46.61 v21.84,46.48
N$1
  Top 0.152: Q4.G 69.53,35.12 69.1,34.68 58.44,34.68 57.88,34.13 | 58.29,34.16 57.85,34.16 57.88,34.13 | 57.88,34.13 R29.2
N$2
  Top 0.152: Q2.G 69.78,47.44 69.6,47.62 67.31,47.62 66.93,48.01 66.23,48.01 R25.2
N$3
  Top 0.152: 65.97,50.42 66.1,50.29 | R24.2 65.88,50.51 65.97,50.42 | Q1.G 69.66,50.86 69.22,50.42 65.97,50.42
N$4
  Top 0.152: Q3.G 69.66,38.92 68.71,37.97 68.2,37.97 67.06,36.83 67.06,35.81 66.64,35.39 59.27,35.39 57.91,36.75 R28.2
N$5
  Top 0.152: Q6.G 67.21,22.8 66.41,23.6 58.81,23.6 58.39,23.18 R34.2
N$6
  Top 0.152: Q5.G 69.66,26.61 68.83,25.78 67.82,25.78 66.36,24.32 59.25,24.32 57.91,25.65 R33.2
N$7
  Top 0.152: U2.P$38 51.93,34.83 52.08,34.98 53.72,34.98 | 53.72,34.98 53.81,34.98 | 53.72,34.98 54.56,34.98 55.12,34.42 55.12,33.67 C33.1
N$8
  Top 0.152: U2.P$43 52.32,37.33 52.7,37.72 52.95,37.72 C32.1
N$9
  Top 0.152: U2.P$48 52.52,39.83 C31.1
N$10
  Top 0.152: U2.P$56 52.09,43.83 52.32,44.07 52.32,47.37 52.45,47.5 52.45,50.79 C27.1
N$11
  Top 0.254: U2.P$27 44.6,30.83 44.96,30.48 44.96,29.47 C20.2
N$12
  Top 0.152: U1.2 19.48,31.92 19.52,31.89 19.52,29.95 U$1.P$1 18.29,28.23 C46.1
N$13
  Top 0.152: U2.P$33 49.86,32.33 46.67,29.15 46.67,27.81 46.51,27.65 45.43,27.65 44.69,26.91 C28.1 44.69,24.58 R18.2
N$14
  Top 0.152: U2.P$32 49.86,31.83 47.03,29 47.03,27.67 46.49,27.13 C28.2 46.49,24.58 R19.2
N$15
  Top 0.152: U2.P$31 49.87,31.33 48.25,29.72 C29.1 48.25,24.58 R20.2
N$16
  Top 0.152: U2.P$30 49.87,30.83 48.6,29.57 48.6,28.36 50.05,26.91 C29.2 50.05,24.58 R21.2
N$17
  Top 0.152: U1.1 18.98,31.92 U$1.P$2 18.29,30.73 17.02,29.46 17.02,28.1 17.22,27.89 17.23,27.89 C9.1
N$18
  Top 0.203: C16.2 C13.2 41.29,37.83 U2.P$13
N$19  (via drill 0.35)
  Top 0.203: 15.41,51.63 C10.2 | C10.2 C11.2 | v13.97,44.32 14.72,45.07 15.88,45.07 16.13,45.32 16.13,46.74 17.08,47.69 17.08,49.84 | C10.2 15.36,51.57 17.08,49.84 | U3.5 17.08,49.84
  Bottom 0.203: v13.97,44.32 12.7,43.05 12.7,38.75 S2.2
  other vias: 12.71,38.73
N$20
  Top 0.203: C17.2 C14.2 40.58,32.83 U2.P$23 44.65,32.83 44.83,33.02 44.83,38.61 44.6,38.83 U2.P$11
N$21
  Top 0.152: U2.P$7 42.81,40.83 41.32,42.32 41.05,42.32 40.36,43.02 40.36,43.16 40.2,43.32 40.18,43.32 R11.1
N$22
  Top 0.203: X1.VBUS 14.32,50.2 14.67,49.84 U3.1 16.32,49.84 16.64,49.53 16.64,48.39 16.2,47.95 U3.3 15.71,46.33 C8.2
N$23
  Top 0.152: C35.1 52.95,42.79 51.99,41.83 U2.P$52
N$24
  Top 0.152: U2.P$49 51.93,40.33 52.17,40.58 52.17,41.01 52.98,41.82 54.02,41.82 54.37,42.17 55.26,42.17 55.43,42.34 55.43,45.97 R17.2
N$25
  Top 0.152: U2.P$9 42.73,39.83 42.66,39.77 42.16,39.77 41.59,40.33 41.59,41.4 41.43,41.56 40.98,41.56 40.26,42.29 R10.1
N$26
  Top 0.152: S3.3 37.93,58.15 R3.1
N$27
  Top 0.152: 51.18,41.27 U2.P$51 52,41.33 52.84,42.17 53.87,42.17 C35.2
  Top 0.203: U2.P$51 50.22,41.33 50.04,41.15 50.35,40.83 U2.P$50 | 49.36,46.65 49.66,46.95 | 49.36,46.65 49.17,46.46 | D4.C 49.66,46.95 | 49.66,46.95 49.36,46.65
  Top 0.305: 50.04,41.15 48.51,42.67 48.51,45.8 49.17,46.46 L2.1
N$30
  Top 0.152: R12.2 42.93,44.53 U2.P$1
N$31
  Top 0.152: U2.P$2 42.77,43.33 41.4,44.7 41.4,45.58 C18.2 C15.2
N$32
  Top 0.152: C15.1 R9.2
N$33
  Top 0.152: U2.P$3 42.76,42.83 40.44,45.16 38.91,45.16 38.74,45.32 38.74,45.34 38.62,45.47 38.62,46.55 38.61,46.56 38.61,46.74 37.66,47.69 R5.1 R4.2
N$34
  Top 0.152: L1.1 20.45,28.28 21,28.83 21,30.35 C12.1
  Top 0.203: 20.48,31.5 U1.4 | 20.48,31.5 20.48,31.37 C12.1 | 20.37,31.13 20.48,31.5
N$35
  Top 0.152: 23.91,52.23 23.95,52.18 | 23.91,52.23 R6.2 | D1.G 24.02,52.34 23.91,52.23
N$36
  Top 0.152: D1.B 24.08,53.84 R8.2
N$39  (via drill 0.3)
  Top 0.152: D1.R 29.22,52.34 v29.34,52.45 | v25.02,50.55 R7.2
  Bottom 0.152: v29.34,52.45 26.92,52.45 v25.02,50.55
NP1RX  (via drill 0.3)
  Top 0.152: U1.26 27.33,37.93 27.65,37.93 27.81,38.09 27.81,38.61 28.7,39.5 29.72,39.5 v29.84,39.37 | J4.3 29.2,15.76 v29.46,15.49
  Bottom 0.152: v29.84,39.37 31.5,37.72 31.5,26.04 29.46,24 v29.46,15.49
NP1TX  (via drill 0.3)
  Top 0.152: U1.25 27.93,37.33 27.93,37.69 28.47,38.24 28.79,38.24 v29.02,38.47 | v28.07,15.49 28.07,17.09 J4.4
  Bottom 0.152: v29.02,38.47 29.09,38.47 30.35,37.21 30.35,26.54 28.32,24.51 28.32,15.75 v28.07,15.49
NP2RX  (via drill 0.3)
  Top 0.152: U1.64 18.6,33.33 19.17,33.91 19.17,34.28 v19.39,34.51 | v21.08,15.62 20.7,15.62 20.32,16 J5.3
  Bottom 0.152: v21.08,15.62 18.41,18.29 18.41,33.53 v19.39,34.51
NP2TX  (via drill 0.3)
  Top 0.152: J5.4 19.31,16.01 v18.92,15.62 | U1.63 18.59,33.83 18.8,34.04 18.8,34.08 18.81,34.09 18.81,35.07 v19.05,35.31
  Bottom 0.152: v18.92,15.62 18.8,15.62 17.27,17.14 17.27,33.53 v19.05,35.31
OCTW  (via drill 0.3)
  Top 0.152: U2.P$5 42.81,41.83 42.57,42.08 42.57,42.53 41.28,43.82 40.92,43.82 v40.61,44.13 | U1.43 21.48,45.32 20.57,46.23 v20.57,47.24
  Bottom 0.152: v40.61,44.13 38.93,44.13 38.35,44.7 37.83,44.7 37.8,44.73 37.26,44.73 37.24,44.7 36.58,44.7 36.07,45.21 36.07,51.31 35.05,52.32 30.99,52.32 28.19,49.53 22.86,49.53 v20.57,47.24
PHASE-U
  Top 0.152: U2.P$46 52.31,38.83 52.45,38.98 53.7,38.98 54.2,39.48 54.2,39.72 C31.2 54.75,40.65 56.14,42.04 56.14,43.32 62.29,49.47 67.88,49.47 68.07,49.28 69.44,49.28 Q2.D@2 | R26.2 67.06,43.43 67.94,44.32 69.5,44.32 Q2.D@4
  pour Top (no thermals): 70.23,50.8 70.23,54.23 71.75,54.23 71.75,51.05 72.9,49.91 77.98,49.91 79.38,48.51 79.38,44.7 77.98,43.31 68.45,43.31 67.69,44.07 67.69,44.7 67.94,44.96 72.01,44.96 72.26,45.21 72.26,47.37 71.5,48.13 67.94,48.13 67.69,48.39 67.69,49.28 68.33,49.91 69.34,49.91
PHASE-V  (via drill 0.3)
  Top 0.152: v62.61,30.73 66.67,30.73 67.82,31.88 69.44,31.88 Q4.D@4 | Q4.D@2 68.73,36.07 68.2,36.07 67.17,35.04 59.12,35.04 56.82,37.34 C32.2 54.36,36.57 54.36,36.48 53.99,36.1 52.67,36.1 52.44,36.33 U2.P$41
  Bottom 0.152: R31.2 66.23,19.75 60.45,25.53 60.45,28.57 v62.61,30.73
  other vias: 66.23,19.56
  pour Top (no thermals): 70.23,38.48 70.23,41.91 71.75,41.91 71.75,38.73 72.9,37.59 77.98,37.59 79.38,36.2 79.38,32.38 77.98,30.99 68.45,30.99 67.69,31.75 67.69,32.38 67.94,32.64 72.01,32.64 72.26,32.89 72.26,35.05 71.5,35.81 67.94,35.81 67.69,36.07 67.69,36.96 68.33,37.59 69.34,37.59
PHASE-W
  Top 0.152: U2.P$36 53.02,33.83 C33.2 53.33,33.29 53.87,32.75 53.87,32.49 56.52,29.85 56.52,29.84 56.88,29.48 56.88,26.18 58.17,24.89 59.1,23.96 67.52,23.96 68.1,24.55 Q6.D@2 | R36.2 66.55,16.76 68.96,19.18 69.06,19.18 Q6.D@4
  pour Top (no thermals): 70.23,26.16 70.23,29.59 71.75,29.59 71.75,26.42 72.9,25.27 77.98,25.27 79.38,23.88 79.38,20.07 77.98,18.67 68.45,18.67 67.69,19.43 67.69,20.07 67.94,20.32 72.01,20.32 72.26,20.57 72.26,22.73 71.5,23.5 67.94,23.5 67.69,23.75 67.69,24.64 68.33,25.27 69.34,25.27
PWMHI1
  Top 0.152: U1.29 27.9,39.33 28.7,40.13 28.7,46.48 J2.3 35.94,48.39 35.94,41.91 36.58,41.27 36.58,37.47 38.93,35.11 41.86,35.11 41.88,35.13 | 41.88,35.13 | U2.P$17 42.59,35.83 41.88,35.13
PWMHI2
  Top 0.152: 42.24,34.48 | 42.24,34.48 42.16,34.4 38.63,34.4 35.87,37.17 35.87,40.98 35.23,41.62 35.23,44.02 J2.5 33.27,45.92 31.52,44.17 31.52,40.15 29.26,37.89 28.62,37.89 28.28,37.55 28.28,37.17 27.94,36.83 U1.24 | U2.P$19 42.59,34.83 42.24,34.48
PWMHI3
  Top 0.152: U1.23 28.71,36.33 J2.7 35.15,39.01 35.15,36.88 38.34,33.69 42.45,33.69 42.6,33.83 U2.P$21
PWMLO1  (via drill 0.3)
  Top 0.152: v29.31,44.58 33.25,48.51 J2.4 35.59,46.2 35.59,41.76 36.22,41.13 36.22,37.32 38.78,34.76 42.01,34.76 42.24,34.98 | U1.19 26.74,34.33 v26.4,34.67 | 42.24,34.98 | U2.P$18 42.59,35.33 42.24,34.98
  Bottom 0.152: v29.31,44.58 29.31,44.55 26.92,42.16 26.92,35.19 v26.4,34.67
PWMLO2  (via drill 0.3)
  Top 0.152: J2.6 34.87,41.83 34.87,41.47 35.51,40.83 35.51,37.02 38.49,34.05 42.3,34.05 42.59,34.33 U2.P$20 | J2.6 33.25,43.43 | U1.18 25.98,33.83 v25.65,34.16 | J2.6 33.15,43.43 31.88,42.16 31.88,40 29.21,37.34 28.89,37.34 v28.86,37.3
  Bottom 0.152: v25.65,34.16 26.04,33.78 26.54,33.78 27.3,34.54 27.3,35.69 28.86,37.24 v28.86,37.3
PWMLO3  (via drill 0.3)
  Top 0.152: J2.8 34.8,36.83 34.8,36.73 38.19,33.33 U2.P$22 | J2.8 32.51,38.35 | U1.17 25.09,33.33 v24.89,33.53 | J2.8 31.62,38.35 v29.39,36.12
  Bottom 0.152: v24.89,33.53 24.95,33.53 25.05,33.43 26.69,33.43 27.05,33.78 v29.39,36.12
RESET  (via drill 0.3)
  Top 0.152: U1.52 19.14,39.33 v19.18,39.37
  Bottom 0.152: v19.18,39.37 19.05,39.37 15.11,35.43 | 15.11,35.43 12.45,32.77 12.45,30.48 J1.2 12.06,28.45 12.45,28.07 12.45,25.96 S1.P$2 10.69,23.89 | R1.2 15.11,35.43
  other vias: 12.06,30.1 14.99,35.55 10.38,23.89
SHNT-V-HI  (via drill 0.35)
  Bottom 0.152: R18.1 45.02,22.67 46.48,24.13 55.63,24.13 58.32,26.82 58.32,30.38 59.44,31.5 59.44,33.08 R30.SB
  other vias: 44.7,22.67 59.37,33.15
SHNT-V-LO  (via drill 0.35)
  Bottom 0.152: R19.1 46.8,22.67 47.75,23.62 55.63,23.62 58.67,26.67 58.67,29.97 60.2,31.5 60.2,38.92 R30.SA
  other vias: 46.48,22.67 59.37,39.75
SHNT-W-HI  (via drill 0.35)
  Bottom 0.152: R20.1 48.26,22.35 48.77,21.84 50.54,21.84 51.61,22.91 58.56,22.91 R35.SB
  other vias: 59.37,22.1 48.26,22.67
SHNT-W-LO  (via drill 0.35)
  Bottom 0.152: R21.1 50.87,22.67 51.46,23.27 55.77,23.27 59.03,26.52 59.03,28.36 R35.SA
  other vias: 50.04,22.67 59.37,28.7
SL-V
  Top 0.152: R30.B 62.87,32.51 61.34,32.51 | 61.34,32.51 60.8,32.51 | U2.P$39 52.61,35.33 52.66,35.39 56.05,35.39 56.26,35.18 56.53,34.91 56.53,31.66 56.92,31.27 60.1,31.27 61.34,32.51
  Top 0.203: R30.B 63.75,32.89
  Top 1.27: Q4.S@1 Q4.S@2 66.91,33.77 66.04,32.89 63.75,32.89
SL-W
  Top 0.152: U2.P$34 52.25,32.83 52.67,32.42 52.94,32.42 55.81,29.55 56.17,29.18 56.17,21.22 57.05,20.35 58.95,20.35 59.21,20.6 59.93,20.6 60.1,20.76 60.1,20.98 60.71,21.59 61.47,21.59 61.72,21.34 | 61.72,21.34 61.21,21.34 | 61.72,21.34 62.74,21.34 R35.B
  Top 1.27: Q6.S@1 Q6.S@2 64.15,21.45 R35.B
SPI_CSN  (via drill 0.3)
  Top 0.152: J6.5 21.31,56.16 21.59,55.88 26.42,55.88 27.08,55.22 27.08,54.84 27.04,54.8 27.04,46.7 v26.83,46.48 | v26.92,31.65 26.51,31.65 25.98,32.18 U1.15
  Bottom 0.152: v26.83,46.48 26.83,44.85 23.77,41.8 23.77,33.13 24.75,32.16 26.42,32.16 v26.92,31.65
SPI_MISO  (via drill 0.3)
  Top 0.152: v26.67,30.79 26.32,30.79 26.24,30.71 25.73,30.71 24.98,31.46 U1.13 | v25.65,47.75 24.64,47.75 22.86,49.53 22.86,55.12 22.69,55.12 22.68,55.13 20.56,55.13 19.3,56.13 J6.3
  Bottom 0.152: v26.67,30.79 26.32,30.79 26.24,30.71 25.18,30.71 23.06,32.83 23.06,42.1 25.68,44.72 25.68,47.72 v25.65,47.75
SPI_MOSI  (via drill 0.3)
  Top 0.152: U1.16 27.11,32.58 v27.18,32.51 | v27.69,46.48 27.39,46.77 27.39,54.65 27.43,54.69 27.43,55.37 26.57,56.24 23.52,56.24 22.81,56.95 J6.6
  Bottom 0.152: v27.18,32.51 24.89,32.51 24.13,33.27 24.13,41.66 27.94,45.47 27.94,46.23 v27.69,46.48
SPI_SCK  (via drill 0.3)
  Top 0.152: U1.14 25.48,31.82 v25.99,31.32 | v26.39,47.27 26.39,48.24 26.67,48.51 26.67,55.12 26.27,55.52 20.93,55.52 20.32,56.13 J6.4
  Bottom 0.152: v25.99,31.32 25.08,31.32 23.42,32.98 23.42,41.95 26.04,44.57 26.04,46.91 v26.39,47.27
STLB
  Top 0.152: R8.1 21.59,54.1 19.81,52.32 19.81,46.49 20.98,45.32 U1.44
SWCLK
  Top 0.152: U1.57 17.91,36.83 17.53,36.45 14.35,36.45 13.97,36.07 13.97,34.42 12.45,32.89 12.45,31.24 13.46,30.23 J1.4
SWDIO  (via drill 0.3)
  Top 0.152: v16.26,33.4 16.26,32 14.61,30.35 J1.6 | U1.58 18.55,36.33 18.81,36.59 18.81,36.72 18.92,36.83 19.3,36.83 v19.43,36.96
  Bottom 0.152: v19.43,36.96 18.41,36.96 17.65,36.2 17.65,35.63 17.02,34.99 16.96,34.99 16.26,34.29 v16.26,33.4
SWO  (via drill 0.3)
  Top 0.152: U1.59 18.75,35.83 18.81,35.89 19.04,35.89 v19.3,36.15
  Bottom 0.152: v19.3,36.15 19,36.15 16.89,34.04 16.89,29.84 16.51,29.46 15.37,29.46 J1.5
  other vias: 14.61,28.83
USBDM  (via drill 0.3)
  Top 0.203: U1.45 20.48,41.11 v20.95,40.64 | v10.91,49.49 13.1,49.49 X1.D-
  Bottom 0.203: v20.95,40.64 20.47,41.12 20.47,41.19 12.61,49.05 11.37,49.05 11.17,49.25 11.15,49.25 v10.91,49.49
USBDP  (via drill 0.3)
  Top 0.203: X1.D+ 11.18,48.9 v10.92,48.64 | U1.46 19.98,40.47 v20.07,40.39
  Bottom 0.203: v10.92,48.64 12.45,48.64 20.07,41.02 v20.07,40.39
V-U  (via drill 0.3)
  Top 0.152: U1.10 23.48,32.14 23.63,32 23.63,31.24 24.13,30.73 24.14,30.73 25.61,29.26 30.43,29.26 31.5,28.19 31.5,27.43 J3.5 34.92,25.65 37.97,22.61 v38.61,22.61 39.37,23.37 D7.A | C39.1 63.12,42.16 v63.25,42.04
  Top 0.203: R26.1 R27.2 62.06,43.33 C39.1
  Bottom 0.152: v63.25,42.04 63.25,41.53 60.55,38.84 60.55,29.18 60.07,28.7 60.07,27.06 59.11,26.1 59.11,23.56 60.07,22.61 60.07,21.84 59.18,20.95 40.26,20.95 v38.61,22.61
V-V  (via drill 0.3)
  Top 0.152: U1.9 22.98,32.13 23.27,31.85 23.27,31.09 23.98,30.38 23.99,30.38 25.46,28.91 30.28,28.91 31.12,28.07 31.12,28.06 31.14,28.04 31.14,27.29 31.88,26.55 31.88,24.51 J3.6 35.05,23.11 36.45,21.72 v38.61,21.72 38.86,21.97 D2.A | C41.1 v64.01,18.29
  Top 0.203: C41.1 62.83,19.46 R32.2 R31.1
  Bottom 0.152: v64.01,18.29 60.83,18.29 58.52,20.6 39.73,20.6 v38.61,21.72
V-VCC  (via drill 0.3)
  Top 0.152: C45.1 v56.39,15.49 | D5.A 39.4,19.18 v38.61,19.97 36.48,19.97 34.54,18.03 J3.8 32,19.3 32,21.34 31.17,22.18 31.17,26.25 30.43,26.99 30.43,27.67 30.13,27.96 26.44,27.96 v26.21,27.74 | v22.81,27.99 22.05,27.99 21.44,28.6 21.44,31.27 21.4,31.31 21.13,31.58 21.13,31.96 20.98,32.1 U1.5
  Top 0.203: R38.1 R39.2 55.21,16.66 C45.1
  Bottom 0.152: v56.39,15.49 56.39,18.29 54.79,19.89 38.69,19.89 v38.61,19.97 | v26.21,27.74 23.07,27.74 v22.81,27.99
V-W  (via drill 0.3)
  Top 0.152: C43.1 v63.88,15.49 | D3.A 38.86,20.57 v38.61,20.83 35.94,20.83 35.69,20.57 J3.7 31.52,22.32 31.52,26.4 30.79,27.14 30.79,27.81 30.28,28.32 v25.65,28.32 | U1.6 21.48,31.73 21.8,31.41 21.8,28.75 21.97,28.57 23.37,28.57 v23.62,28.32
  Top 0.203: C43.1 62.83,16.66 R37.2 R36.1
  Bottom 0.152: v63.88,15.49 60.96,15.49 56.21,20.24 39.19,20.24 v38.61,20.83 | v23.62,28.32 v25.65,28.32
VCC
  pour Top (rank 2): 48.39,61.98 48.39,42.93 50.42,40.89 50.42,29.97 43.69,29.97 43.69,12.19 99.06,12.19 99.06,61.98
VDDCORE
  Top 0.203: U1.53 16.96,38.83 C7.1 15.2,38.9 C5.2

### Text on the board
tPlace: VCC | GND | SPI | < no - go > | mkbldcdriver v0.31 | GND | FAULT | HI1 | U | LO1 | HI2 | LO2 | drv | HI3 | LO3 | GND | V | usb | 3V3 | I-V | I-W | V-U | V-V | W | V-W | NP2 | NP1 | V-VCC | VCC | VCC | GND
bPlace: "wow" / - Owen Wilson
